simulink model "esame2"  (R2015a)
settings: Solver=ode45  StartTime=0.0  StopTime=20  MaxStep=1e-3  RelTol=1e-3
libraries: simulink_extras x2, simulink x2

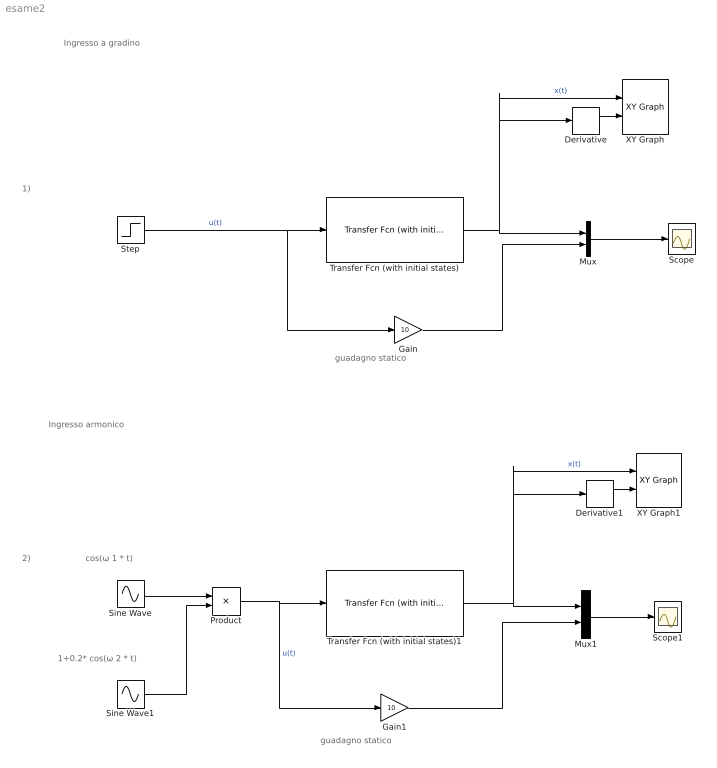
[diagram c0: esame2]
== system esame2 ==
  note: Ingresso a gradino
  note: cos(ω 1 * t)
  note: guadagno statico
  note: 1)
  note: 2)
  note: 1+0.2* cos(ω 2 * t)
  note: guadagno statico
  note: Ingresso armonico
  Derivative : Derivative
  Derivative1 : Derivative
  Gain : Gain  Gain=10
  Gain1 : Gain  Gain=10
  Mux : Mux  Inputs=2
  Mux1 : Mux  Inputs=2
  Product : Product
  Scope : Scope
  Scope1 : Scope
  Sine Wave : Sin  Frequency=5  Phase=pi/2  SampleTime=0
  Sine Wave1 : Sin  Amplitude=0.2  Bias=1  Phase=pi/2  SampleTime=0
  Step : Step  After=5  SampleTime=0
  Transfer Fcn (with initial states) : simulink_extras/Additional Linear/Transfer Fcn (with initial states)  N=[1000]  D="[1  2  100]"  X0=0
  Transfer Fcn (with initial states)1 : simulink_extras/Additional Linear/Transfer Fcn (with initial states)  N=[1000]  D="[1  2  100]"  X0=0
  XY Graph : simulink/Sinks/XY Graph  xmin=-1  xmax=500  ymin=-500  ymax=500  st=-1
  XY Graph1 : simulink/Sinks/XY Graph  xmin=-100  xmax=100  ymin=-200  ymax=200  st=-1
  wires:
  Step/1 -> Gain/1, Transfer Fcn (with initial states)/1  "u(t)"
  Transfer Fcn (with initial states)/1 -> Derivative/1, XY Graph/1, Mux/1  "x(t)"
  Mux/1 -> Scope/1
  Gain/1 -> Mux/2
  Mux1/1 -> Scope1/1
  Gain1/1 -> Mux1/2
  Sine Wave/1 -> Product/1
  Sine Wave1/1 -> Product/2
  Product/1 -> Gain1/1, Transfer Fcn (with initial states)1/1  "u(t)"
  Derivative/1 -> XY Graph/2
  Transfer Fcn (with initial states)1/1 -> XY Graph1/1, Derivative1/1, Mux1/1  "x(t)"
  Derivative1/1 -> XY Graph1/2
